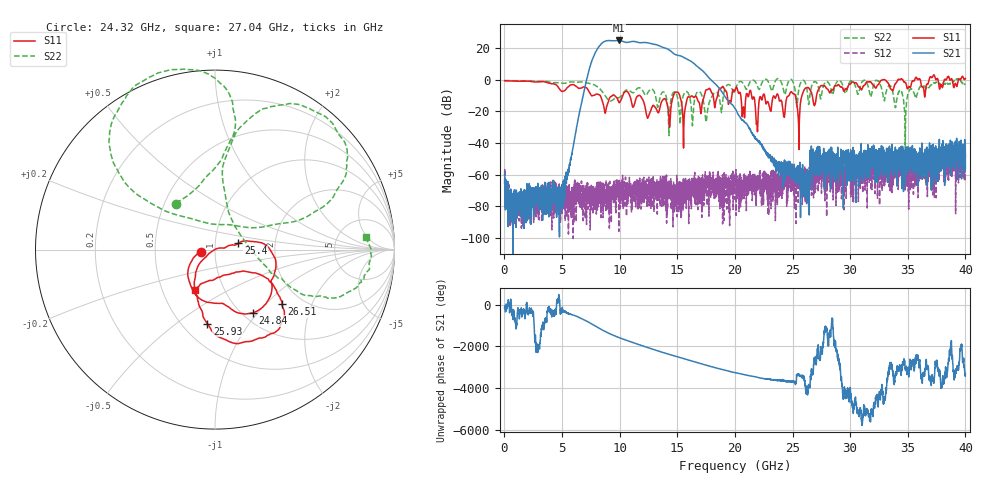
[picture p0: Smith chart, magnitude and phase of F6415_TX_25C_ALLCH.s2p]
!Keysight Technologies,N5245B,MY52451815,A.15.70.20
!Date: Thursday, April 18, 2024 10:02:07
!Correction: S33(C  2-Port  )
!S43(C  2-Port  )
!S34(C  2-Port  )
!S44(C  2-Port  )
!S2P File: Measurements: S33, S43, S34, S44:
# Hz S  RI  R 50
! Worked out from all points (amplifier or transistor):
!   4000 points, 10 MHz to 40 GHz, reference 50 ohm
!   highest |S21| = 24.8 dB at 9.9 GHz (marker M1)
!   |S21| within 3 dB of that: 8.297 GHz to 13.32 GHz (5.019 GHz wide, 46.4 % of centre)
!   unconditionally stable (mu >= 1): start of sweep to 22.5 GHz; 24.92 GHz to 32.84 GHz; 33 GHz to 34.13 GHz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
!   at 6.67 GHz: K = 6371.84, MAG = -7.7 dB, |S12| = -81.6 dB
!   at 20.01 GHz: K = 5158.94, MAG = -16.2 dB, |S12| = -66.1 dB
!   at 40 GHz: K = -7126.23, MSG = -3.3 dB, |S12| = -49.4 dB
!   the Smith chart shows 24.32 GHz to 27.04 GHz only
!   S11 on the Smith chart (normalised r, x): 24.32 GHz: 0.85, -0.02; 24.84 GHz: 1.12, -0.94; 25.4 GHz: 1.29, +0.09; 25.93 GHz: 0.66, -0.65; 26.51 GHz: 1.58, -1.25; 27.04 GHz: 0.73, -0.35
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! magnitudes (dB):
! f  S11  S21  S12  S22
! 10 MHz  -0.7  -60.5  -66.1  -0.5
! 570 MHz  -0.8  -75.8  -87.7  -0.6
! 4.71 GHz  -5.3  -73.1  -74.0  -1.9
! 6.68 GHz  -5.2  -14.6  -64.0  -1.4
! 8.02 GHz  -9.0  18.9  -76.2  -4.3
! 9.9 GHz  -14.0  24.8  -68.8  -11.4
! 13.34 GHz  -20.9  21.7  -66.0  -16.9
! 16.88 GHz  -14.3  7.5  -60.7  -7.5
! 17.52 GHz  -6.4  3.1  -73.8  -26.1
! 20.01 GHz  -6.8  -18.2  -66.1  -6.8
! 21.9 GHz  -27.0  -37.5  -65.1  -3.0
! 22.37 GHz  -12.2  -42.1  -64.5  -1.5
! 24.32 GHz  -21.9  -57.9  -57.5  -9.5
! 24.84 GHz  -7.7  -57.3  -71.3  0.3
! 25.4 GHz  -17.4  -61.4  -60.8  -15.8
! 25.93 GHz  -7.7  -63.3  -63.5  -0.4
! 26.51 GHz  -6.4  -48.4  -58.2  -9.4
! 26.67 GHz  -8.8  -45.1  -68.8  -3.7
! 27.04 GHz  -12.1  -52.8  -59.1  -1.5
! 33.34 GHz  -2.8  -52.3  -52.2  -3.9
! 34.77 GHz  -1.7  -50.9  -70.6  -33.4
! 40 GHz  0.7  -56.0  -49.4  -2.6
